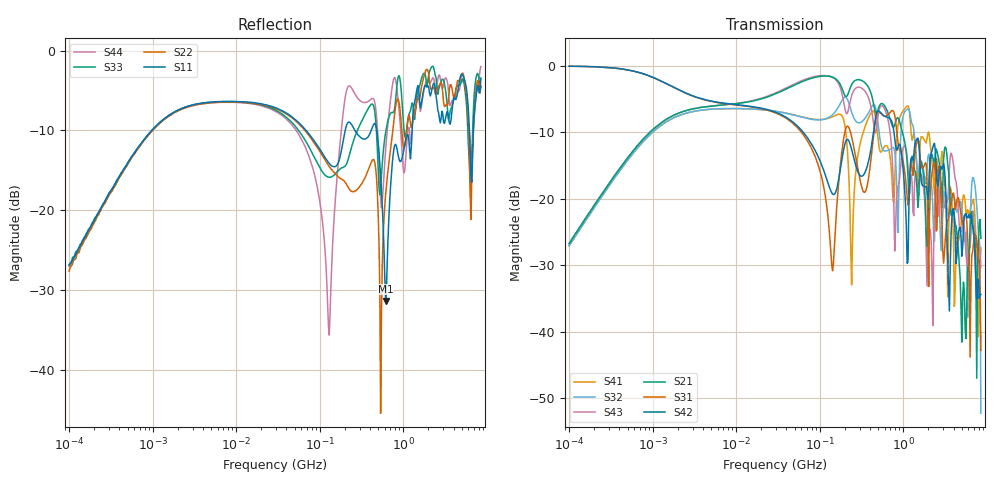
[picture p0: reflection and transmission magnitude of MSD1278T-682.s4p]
# MHz S MA R 50
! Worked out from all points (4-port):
!   498 points, 100 kHz to 8.5 GHz, reference 50 ohm
!   strongest paths, dB at 100 kHz, 1.698 MHz, 29.49 MHz, 500.7 MHz, 8.5 GHz:
!     S42: -0.1, -3.1, -7.0, -6.8, -34.4
!     S31: -0.1, -3.1, -7.1, -6.9, -42.8
!     S21: -26.8, -7.6, -4.2, -6.6, -26.0
!     S43: -26.8, -7.6, -4.1, -7.4, -30.4
!     S32: -27.1, -8.0, -6.9, -8.8, -52.3
!     S41: -27.1, -8.0, -6.9, -11.1, -27.4
!   lowest |S11| = -31.4 dB at 614.9 MHz (marker M1), VSWR 1.06, Z = 48.5 + j2.24 ohm
!   |S11| at or under -10 dB: 263.8 MHz to 413.8 MHz (150.1 MHz wide, 44.3 % of centre); 482.5 MHz to 1.276 GHz (793.6 MHz wide, 90.3 % of centre); 6.197 GHz to 6.912 GHz (715.7 MHz wide, 10.9 % of centre)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
0.1  0.04544 82.3  0.04579 83.0  0.9902 -2.7  0.04413 -97.2
     0.04579 83.0  0.04153 84.1  0.04418 -97.3  0.9903 -2.6
     0.9902 -2.7  0.04418 -97.3  0.04506 83.7  0.0458 82.6
     0.04413 -97.2  0.9903 -2.6  0.0458 82.6  0.04452 85.5
5.827281  0.4779 4.7  0.5009 14.4  0.5288 -16.9  0.4727 -177.5
          0.5009 14.4  0.4729 5.0  0.4731 -177.2  0.532 -16.8
          0.5288 -16.9  0.4731 -177.2  0.4764 5.0  0.5014 14.3
          0.4727 -177.5  0.532 -16.8  0.5014 14.3  0.4726 4.8
142.5721  0.1884 -121.6  0.8201 -27.5  0.02866 -32.0  0.413 43.8
          0.8201 -27.5  0.1764 -92.0  0.4277 63.8  0.1084 -65.8
          0.02866 -32.0  0.4277 63.8  0.1634 -50.4  0.8157 -38.4
          0.413 43.8  0.1084 -65.8  0.8157 -38.4  0.0607 115.9
614.9063  0.02705 121.7  0.4848 -105.9  0.4177 -35.5  0.2503 -53.5
          0.4848 -105.9  0.1247 23.7  0.2281 -78.6  0.4133 -41.6
          0.4177 -35.5  0.2281 -78.6  0.306 -22.3  0.4534 -135.2
          0.2503 -53.5  0.4133 -41.6  0.4534 -135.2  0.2375 -28.9
2209.207  0.575 -168.2  0.2142 149.7  0.1546 128.1  0.1893 92.6
          0.2142 149.7  0.576 180.0  0.1134 70.3  0.2305 136.9
          0.1546 128.1  0.1134 70.3  0.7934 179.8  0.02806 116.7
          0.1893 92.6  0.2305 136.9  0.02806 116.7  0.6629 -172.4
6920.76  0.3232 48.9  0.05425 5.2  0.0452 72.6  0.09906 37.5
         0.05425 5.2  0.3157 -4.0  0.1432 59.2  0.05848 -6.8
         0.0452 72.6  0.1432 59.2  0.4243 36.6  0.07596 12.8
         0.09906 37.5  0.05848 -6.8  0.07596 12.8  0.352 58.6
8500  0.6731 -28.8  0.05029 -86.6  0.007211 -153.8  0.04253 -57.9
      0.05029 -86.6  0.5972 -39.6  0.002425 144.5  0.01905 -141.9
      0.007211 -153.8  0.002425 144.5  0.5913 -41.2  0.03033 -100.3
      0.04253 -57.9  0.01905 -141.9  0.03033 -100.3  0.793 -40.8
